ORGANIZATION_BLOCK MAIN:OB1
TITLE=Semaforo Pedonale
//Simulatore: 16
//Versione:1.0
//Data 02/03/2002
//----- Descrizione del controllo ---------------------------
//Per la sicurezza dei pedoni e degli automobilisti il programma
//deve tenere conto dei seguenti aspetti relativi alla sicurezza:
//  A) La preimpostazione deve essere: verde per il semaforo
//     automobilistico e rosso per il semaforo pedonale in modo da
//     avere  una situazione iniziale sicura.
//  B) Se in seguito alla pressione del pulsante  il programma riceve
//     la richiesta di commutare il semaforo pedonale sul verde
//     allora il semaforo automobilistico commuta sul giallo e poi
//     sul rosso.
//Oltre  ai requisiti di sicurezza vengono di seguito definite le
//fasi dei semafori e quandi esse devono venire avviate:
//
//    1) la fase del giallo per il traffico automobilistico deve
//       durare 2 secondi.
//    2) La fase del rosso per il traffico automobilistico deve
//       durare 16 secondi e contemporaneamente deve iniziare la
//       fase del verde per il traffico pedonale.
//    3) La fase del verde per il traffico pedonale deve durare
//       10 secondi.
//    4) Non appena la fase del verde per il traffico pedonale è
//       terminata il semaforo pedonale deve commutare sul rosso.
//    5) La fase rosso/giallo per il traffico automobilistico deve
//       durare 3 secondi.
//    6) Il ritardo per la successiva richiesta del verde per i
//       pedoni deve durare 1 s.

BEGIN
NETWORK 1 //Rilevamento richiesta del verde per i pedoni
//
LD I0.0
O I0.1
A T36
O M0.0
AN T35
= M0.0

NETWORK 2 //Fase del Verde per le Auto
//
LDN M0.0
= Q0.4

NETWORK 3 //Timer per fase giallo auto
//
LD M0.0
TON T32 +50

NETWORK 4 //Fase del Giallo per le Auto
//
LD M0.0
LDN T32
O T34
ALD
= Q0.3

NETWORK 5 //Fase del Rosso per le Auto
//
LD M0.0
A T32
= Q0.2

NETWORK 6 //Avvio timer per fase Verde pedoni
//
LD Q0.2
TON T33 +100

NETWORK 7 //Fase Verde per Pedoni
//
LD Q0.2
AN T33
= Q0.1

NETWORK 8 //Avvio Timer per ritardo fase giallo per le auto
//
LD M0.0
A T33
TON T34 +50

NETWORK 9 //Fase del Rosso per i pedoni
//
LD M0.0
LDN T32
O T33
ALD
ON M0.0
= Q0.0

NETWORK 10 //Avvio Timer fase Rosso-Giallo per le auto
//
LD M0.0
A T34
TON T35 +50

NETWORK 11 //Avvio Timer per ritardo richiesta Verde
//
LD Q0.4
TON T36 +5

END_ORGANIZATION_BLOCK

